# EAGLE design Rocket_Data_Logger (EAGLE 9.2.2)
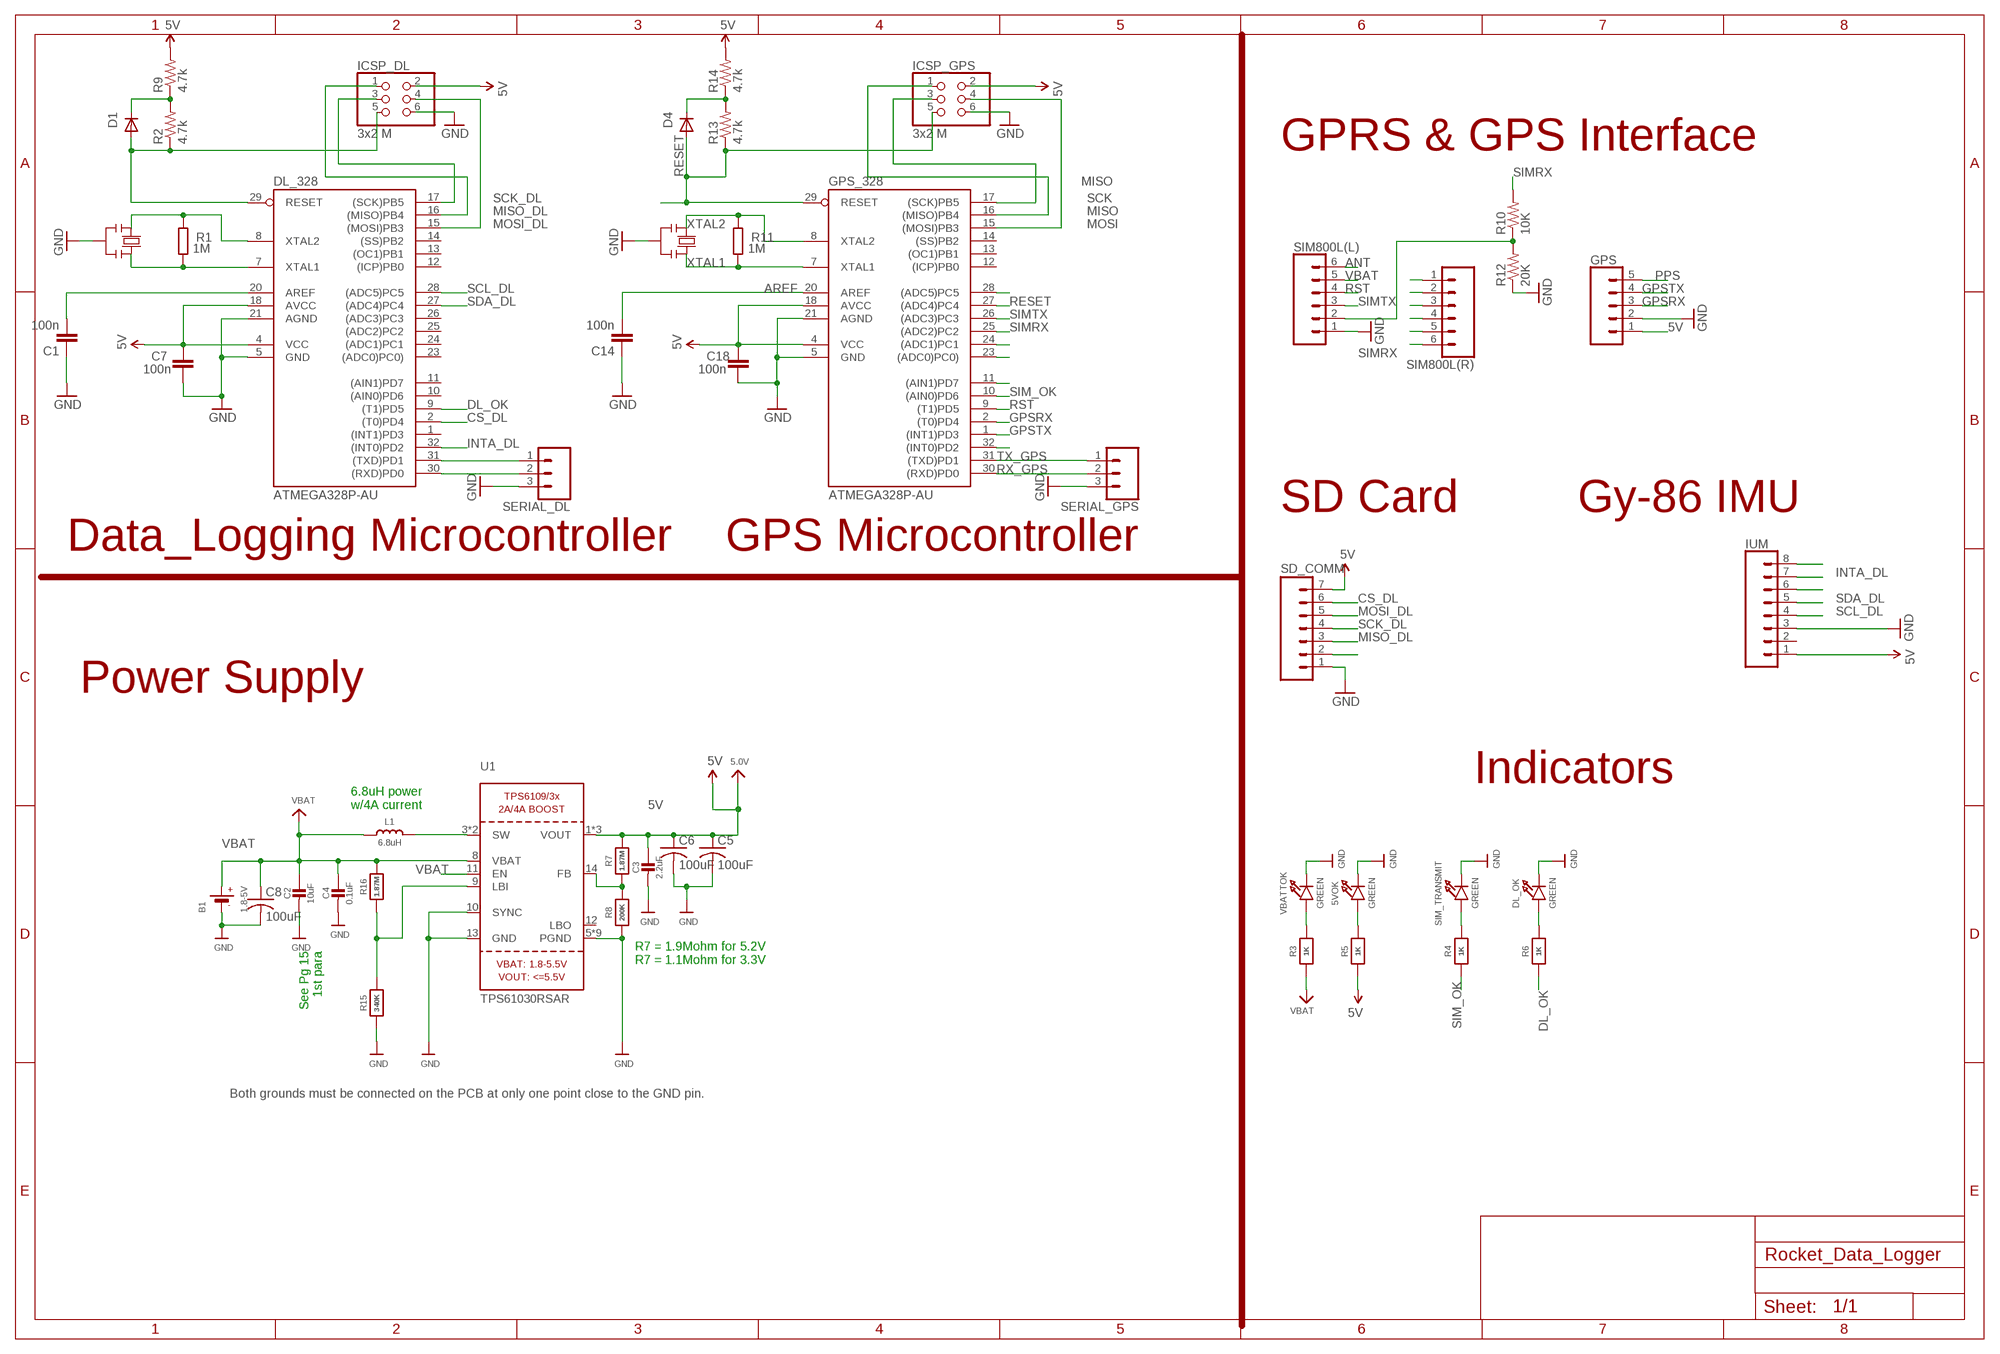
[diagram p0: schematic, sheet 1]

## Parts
5VOK  GREEN  LED0805_NOOUTLINE  [CHIPLED_0805_NOOUTLINE]
B1  1.8-5V  BATTERY  [JSTPH2]
C1  100n  C-EUC0805  [C0805]
C2  10uF  CAP_CERAMIC0805-NOOUTLINE  [0805-NO]
C3  2.2uF  CAP_CERAMIC0805-NOOUTLINE  [0805-NO]
C4  0.1uF  CAP_CERAMIC0805-NOOUTLINE  [0805-NO]
C5  100uF  C-USC1210  [C1210]
C6  100uF  C-USC1210  [C1210]
C7  100n  C-EUC0805  [C0805]
C8  100uF  C-USC1210  [C1210]
C14  100n  C-EUC0805  [C0805]
C18  100n  C-EUC0805  [C0805]
D1  DIODE-MINIMELF  [MINIMELF]
D4  DIODE-MINIMELF  [MINIMELF]
DL_328  ATMEGA328P-AU  [TQFP32-08]
DL_OK  GREEN  LED0805_NOOUTLINE  [CHIPLED_0805_NOOUTLINE]
GPS  CONN_05  [1X05]
GPS_328  ATMEGA328P-AU  [TQFP32-08]
ICSP_DL  3x2 M  PINHD-2X3  [2X03]
ICSP_GPS  3x2 M  PINHD-2X3  [2X03]
IUM  CONN_08"  [1X08]
L1  6.8uH  INDUCTOR-8X8  [INDUCTOR_8X8MM]
R1  1M  R-EU_R0805  [R0805]
R2  4.7k  4.7KOHM1/10W1%(0603)  [0603@1]
R3  1K  RESISTOR0805_NOOUTLINE  [0805-NO]
R4  1K  RESISTOR0805_NOOUTLINE  [0805-NO]
R5  1K  RESISTOR0805_NOOUTLINE  [0805-NO]
R6  1K  RESISTOR0805_NOOUTLINE  [0805-NO]
R7  1.87M  RESISTOR_0805MP  [_0805MP]
R8  200K  RESISTOR0805_NOOUTLINE  [0805-NO]
R9  4.7k  4.7KOHM1/10W1%(0603)  [0603@1]
R10  10K  RESISTOR0805-RES  [0805]
R11  1M  R-EU_R0805  [R0805]
R12  20K  RESISTOR0805-RES  [0805]
R13  4.7k  4.7KOHM1/10W1%(0603)  [0603@1]
R14  4.7k  4.7KOHM1/10W1%(0603)  [0603@1]
R15  340K  RESISTOR_0805MP  [_0805MP]
R16  1.87M  RESISTOR_0805MP  [_0805MP]
SD_COMM  M07  [1X07]
SERIAL_DL  CONN_03  [1X03]
SERIAL_GPS  CONN_03  [1X03]
SIM800L(L)  CONN_06SILK_FEMALE_PTH  [1X06]
SIM800L(R)  CONN_06SILK_FEMALE_PTH  [1X06]
SIM_TRANSMIT  GREEN  LED0805_NOOUTLINE  [CHIPLED_0805_NOOUTLINE]
U1  TPS61030RSAR  VREG_TPS6103X  [PVQFN-16]
VBATTOK  GREEN  LED0805_NOOUTLINE  [CHIPLED_0805_NOOUTLINE]
Y1  RESONATORMU  [RESONATOR]
Y2  RESONATORMU  [RESONATOR]

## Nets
5V: C3.1 C5.1 C6.1 C7.2 C18.2 DL_328.4(VCC) DL_328.18(AVCC) GPS.1 GPS_328.4(VCC) GPS_328.18(AVCC) ICSP_DL.2 ICSP_GPS.2 IUM.1 R5.1 R7.2 R9.2 R14.2 SD_COMM.7 U1.1(VOUT) U1.15(VOUT) U1.16(VOUT) ; supply symbol labelled 5.0V
ANT: SIM800L(L).6
AREF [aref]: C14.2 GPS_328.20(AREF)
CS_DL: DL_328.2((T0)PD4) SD_COMM.6
DL_OK: DL_328.9((T1)PD5) R6.1
FPS_RX: R10.1 R12.2 SIM800L(L).2
GND: 5VOK.C B1.1(-) C1.1 C2.2 C3.2 C4.2 C5.2 C6.2 C7.1 C8.2 C14.1 C18.1 DL_328.5(GND) DL_328.21(AGND) DL_OK.C GPS.2 GPS_328.5(GND) GPS_328.21(AGND) ICSP_DL.6 ICSP_GPS.6 IUM.3 R8.1 R12.1 R15.1 SD_COMM.1 SERIAL_DL.3 SERIAL_GPS.3 SIM800L(L).1 SIM_TRANSMIT.C U1.5(PGND) U1.6(PGND) U1.7(PGND) U1.10(SYNC) U1.13(GND) U1.P$18(PGND) U1.P$19(PGND) U1.P$20(PGND) U1.P$21(PGND) U1.P$22(PGND) U1.THERMAL(PGND) VBATTOK.C Y1.2 Y2.2
GPSRX: GPS.3 GPS_328.2((T0)PD4)
GPSTX: GPS.4 GPS_328.1((INT1)PD3)
INTA_DL: DL_328.32((INT0)PD2) IUM.7
MISO: GPS_328.16((MISO)PB4) ICSP_GPS.1
MISO_DL: DL_328.16((MISO)PB4) ICSP_DL.1 SD_COMM.3
MOSI: GPS_328.15((MOSI)PB3) ICSP_GPS.4
MOSI_DL: DL_328.15((MOSI)PB3) ICSP_DL.4 SD_COMM.5
N$1: D1.C R2.2 R9.1
N$2: DL_328.8(XTAL2) R1.2 Y1.1
N$3: L1.P$2 U1.3(SW) U1.4(SW)
N$4: IUM.6
N$5: D1.A DL_328.29(RESET) ICSP_DL.5 R2.1
N$6: IUM.8
N$7: R15.2 R16.1 U1.9(LBI)
N$9: R7.1 R8.2 U1.14(FB)
N$11: 5VOK.A R5.2
N$12: GPS_328.32((INT0)PD2)
N$13: DL_328.7(XTAL1) R1.1 Y1.3
N$14: C1.2 DL_328.20(AREF)
N$15: DL_328.31((TXD)PD1) SERIAL_DL.1
N$17: GPS_328.11((AIN1)PD7)
N$18: D4.C R13.2 R14.1
N$19: SD_COMM.2
N$20: DL_328.30((RXD)PD0) SERIAL_DL.2
N$21: R3.2 VBATTOK.A
N$22: SIM800L(R).1
N$23: SIM800L(R).2
N$24: SIM800L(R).3
N$25: SIM800L(R).4
N$26: SIM800L(R).5
N$27: SIM800L(R).6
N$28: R4.2 SIM_TRANSMIT.A
N$29: GPS_328.23((ADC0)PC0))
N$30: GPS_328.24((ADC1)PC1)
N$31: DL_OK.A R6.2
N$34: GPS_328.28((ADC5)PC5)
PPS: GPS.5
RESET: D4.A GPS_328.27((ADC4)PC4) GPS_328.29(RESET) ICSP_GPS.5 R13.1
RST: GPS_328.9((T1)PD5) SIM800L(L).4
RX_GPS: GPS_328.30((RXD)PD0) SERIAL_GPS.2
SCK: GPS_328.17((SCK)PB5) ICSP_GPS.3
SCK_DL: DL_328.17((SCK)PB5) ICSP_DL.3 SD_COMM.4
SCL_DL: DL_328.28((ADC5)PC5) IUM.4
SDA_DL: DL_328.27((ADC4)PC4) IUM.5
SIM_OK: GPS_328.10((AIN0)PD6) R4.1
SIMRX: GPS_328.25((ADC2)PC2) R10.2
SIMTX: GPS_328.26((ADC3)PC3) SIM800L(L).3
TX_GPS: GPS_328.31((TXD)PD1) SERIAL_GPS.1
VBAT: B1.2(+) C2.1 C4.1 C8.1 L1.P$1 R3.1 R16.2 SIM800L(L).5 U1.8(VBAT) U1.11(EN)
XTAL1: GPS_328.7(XTAL1) R11.1 Y2.3
XTAL2: GPS_328.8(XTAL2) R11.2 Y2.1
Unconnected: DL_328.1((INT1)PD3) DL_328.10((AIN0)PD6) DL_328.11((AIN1)PD7) DL_328.12((ICP)PB0) DL_328.13((OC1)PB1) DL_328.14((SS)PB2) DL_328.23((ADC0)PC0)) DL_328.24((ADC1)PC1) DL_328.25((ADC2)PC2) DL_328.26((ADC3)PC3) GPS_328.12((ICP)PB0) GPS_328.13((OC1)PB1) GPS_328.14((SS)PB2) IUM.2 U1.12(LBO)

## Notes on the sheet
- GPRS & GPS Interface
- SD Card | Gy-86 IMU
- Data_Logging Microcontroller | GPS Microcontroller
- Power Supply
- Indicators
- 6.8uH power
  w/4A current
- See Pg 15
  1st para
- R7 = 1.9Mohm for 5.2V
  R7 = 1.1Mohm for 3.3V
- Both grounds must be connected on the PCB at only one point close to the GND pin.

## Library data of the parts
5VOK DL_OK SIM_TRANSMIT VBATTOK = microbuilder:LED: LED
B1 = microbuilder:BATTERY: CR1220 SMT - Digikey: 3001K-ND
C1 C7 C14 C18 = SmartPrj:C-EU: CAPACITOR, European symbol
C2-C4 = microbuilder:CAP_CERAMIC: Ceramic Capacitors
C5 C6 C8 = rcl:C-US: CAPACITOR, American symbol
D1 D4 = diode:DIODE-: DIODE
DL_328 GPS_328 = SmartPrj:ATMEGA328P-: MICROCONTROLLER 4 Kbytes FLASH 128 bytes SRAM 256 bytes EEPROM UART 6-channel 10 bit ADC
GPS = SparkFun-Connectors:CONN_05: Multi connection point. Often used as Generic Header-pin footprint for 0.1 inch spaced/style header connections On any of the 0.1 inch spaced packages, you can populate with these: Break Away Headers - Straight (PRT-00116) Break Away Male Headers - Right Angle (PRT-00553) Female Headers (PRT-00115)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
ICSP_DL ICSP_GPS = SmartPrj:PINHD-2X3: PIN HEADER
IUM = SparkFun-Connectors:CONN_08: Multi connection point. Often used as Generic Header-pin footprint for 0.1 inch spaced/style header connections On any of the 0.1 inch spaced packages, you can populate with these: Break Away Headers - Straight (PRT-00116) Break Away Male Headers - Right Angle (PRT-00553) Female Headers (PRT-00115)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; PROD_ID: CONN-08438
L1 = microbuilder:INDUCTOR: Inductors
R1 R11 = SmartPrj:R-EU_: RESISTOR, European symbol
R2 R9 R13 R14 = SparkFun-Resistors:4.7KOHM1/10W1%(0603): RES-07857; PROD_ID: RES-07857
R3-R8 R15 R16 = microbuilder:RESISTOR: Resistors
R10 R12 = SparkFun:RESISTOR: Resistor
SD_COMM = SparkFun-Connectors:M07: Header 7 Standard 7-pin 0.1" header. Use with straight break away headers (SKU : PRT-00116), right angle break away headers (PRT-00553), swiss pins (PRT-00743), machine pins (PRT-00117), and female headers (PRT-00115). NOTES ON THE VARIANTS LOCK and LOCK_LONGPADS... This footprint was designed to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
SERIAL_DL SERIAL_GPS = SparkFun-Connectors:CONN_03: Multi connection point. Often used as Generic Header-pin footprint for 0.1 inch spaced/style header connections On any of the 0.1 inch spaced packages, you can populate with these: Break Away Headers - Straight (PRT-00116) Break Away Male Headers - Right Angle (PRT-00553) Female Headers (PRT-00115)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
SIM800L(L) SIM800L(R) = SparkFun-Connectors:CONN_06: Multi connection point. Often used as Generic Header-pin footprint for 0.1 inch spaced/style header connections On any of the 0.1 inch spaced packages, you can populate with these: Break Away Headers - Straight (PRT-00116) Break Away Male Headers - Right Angle (PRT-00553) Female Headers (PRT-00115)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; PROD_ID: CONN-08437
U1 = microbuilder:VREG_TPS6103X: TPS6103x 4A Boost - 1.8-5.5V Input, Adjustable Output to 5.5V
Y1 Y2 = SmartPrj:RESONATOR

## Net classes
0 default: width 0.152 mm, drill 0.305 mm, clearance 0.152 mm
3 usbvcc: width 0.508 mm, drill 0.61 mm, clearance 0.254 mm
4 aref: width 0.406 mm, drill 0.61 mm, clearance 0.254 mm

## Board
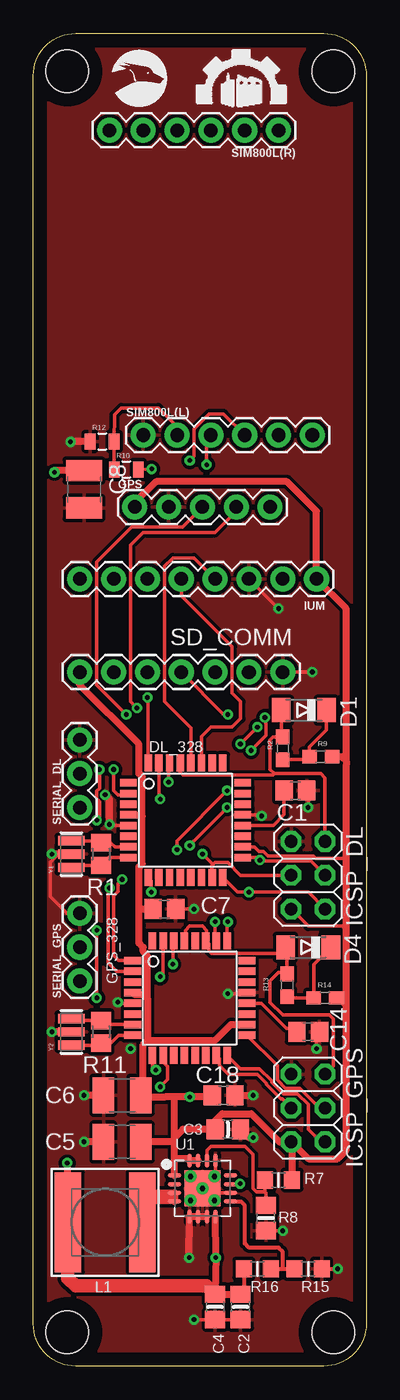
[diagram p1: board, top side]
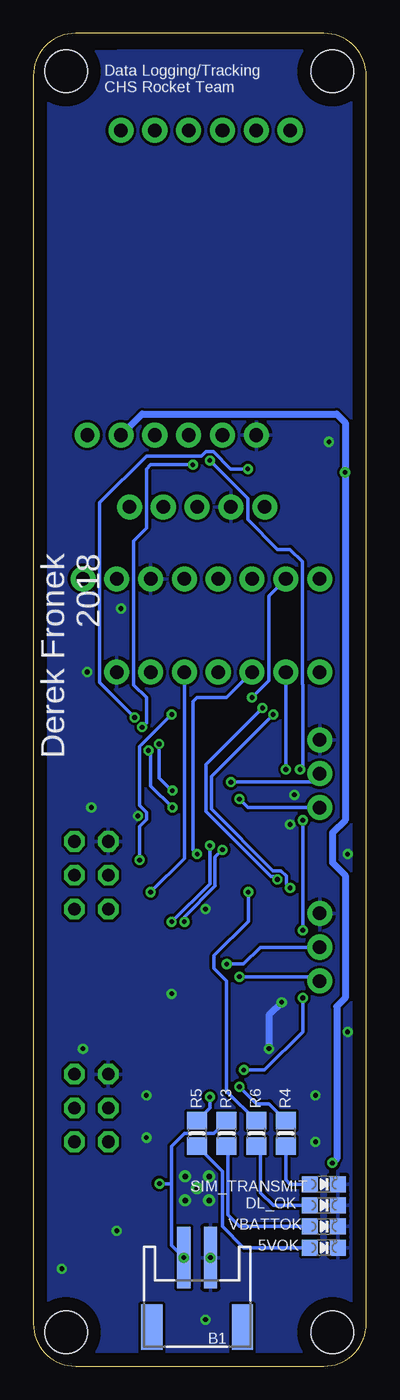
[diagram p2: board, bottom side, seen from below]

Size 25 x 99.99 mm. Coordinates in mm from the lower left corner, seen from the top.
Outline: 25,96.81 25,3.17 arc-90 21.82,0 3.17,0 arc-90 0,3.17 0,96.81 arc-90 3.17,99.99 21.82,99.99 arc-90 25,96.81
Copper layers (1*16): Top 0.035mm / dielectric 1.5mm / Bottom 0.035mm
Design rules "default": minimum track width 6mil, minimum drill 0.35mm, track to track 6mil, track to pad 6mil, pad to pad 6mil, via to via 6mil, smd to smd 6mil, copper to edge 40mil, drill to drill 6mil, minimum pad ring 10mil, minimum via ring 8mil, stop-mask expansion 4mil, vias tented up to drill 0mil, thermal gap 10mil
Holes 3.2 mm at 22.54,97.16 2.54,2.54 2.54,97.16 22.54,2.54

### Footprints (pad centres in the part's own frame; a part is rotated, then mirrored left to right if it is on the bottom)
CHIPLED_0805_NOOUTLINE = smd 1.2 x 1.2: A 0,-1.05; C 0,1.05
JSTPH2 = smd 1 x 4.6: 1 -1,-3.7; 2 1,-3.7 | smd 1.6 x 3.4: NC1 -3.4,1.5; NC2 3.4,1.5
C0805 = smd 1.3 x 1.5: 1 -0.85,0; 2 0.85,0
0805-NO = smd 1.3 x 1.5: 1 -0.95,0; 2 0.95,0
C1210 = smd 1.6 x 2.7: 1 -1.4,0; 2 1.4,0
MINIMELF = smd 1.4 x 1.8: A 1.7,0; C -1.7,0
TQFP32-08 = smd 1.27 x 0.559: 1 -4.293,2.8; 2 -4.293,2; 3 -4.293,1.2; 4 -4.293,0.4; 5 -4.293,-0.4; 6 -4.293,-1.2; 7 -4.293,-2; 8 -4.293,-2.8; 17 4.293,-2.8; 18 4.293,-2; 19 4.293,-1.2; 20 4.293,-0.4; 21 4.293,0.4; 22 4.293,1.2; 23 4.293,2; 24 4.293,2.8 | smd 0.559 x 1.27: 9 -2.8,-4.293; 10 -2,-4.293; 11 -1.2,-4.293; 12 -0.4,-4.293; 13 0.4,-4.293; 14 1.2,-4.293; 15 2,-4.293; 16 2.8,-4.293; 25 2.8,4.293; 26 2,4.293; 27 1.2,4.293; 28 0.4,4.293; 29 -0.4,4.293; 30 -1.2,4.293; 31 -2,4.293; 32 -2.8,4.293
1X05 = drill 1.016 pad 1.88: 1 0,0; 2 2.54,0; 3 5.08,0; 4 7.62,0; 5 10.16,0
2X03 = drill 0.95 pad 1.55 octagon: 1 -2.54,-1.27; 2 -2.54,1.27; 3 0,-1.27; 4 0,1.27; 5 2.54,-1.27; 6 2.54,1.27
1X08 = drill 1.016 pad 1.88: 1 0,0; 2 2.54,0; 3 5.08,0; 4 7.62,0; 5 10.16,0; 6 12.7,0; 7 15.24,0; 8 17.78,0
INDUCTOR_8X8MM = smd 2 x 7.5: P$1 -2.8,0; P$2 2.8,0
R0805 = smd 1.3 x 1.5: 1 -0.85,0; 2 0.85,0
0603@1 = smd 1.1 x 1: 1 -0.85,0; 2 0.85,0
_0805MP = smd 1.2 x 1.3: 1 -1.016,0; 2 1.016,0
0805 = smd 0.8 x 1.2: 1 -0.9,0; 2 0.9,0
1X07 = drill 1.016 pad 1.88: 1 0,0; 2 2.54,0; 3 5.08,0; 4 7.62,0; 5 10.16,0; 6 12.7,0; 7 15.24,0
1X03 = drill 1.016 pad 1.88: 1 0,0; 2 2.54,0; 3 5.08,0
1X06 = drill 1.016 pad 1.88: 1 0,0; 2 2.54,0; 3 5.08,0; 4 7.62,0; 5 10.16,0; 6 12.7,0
PVQFN-16 = smd 1.05 x 0.35: 1 -2.1,0.975; 2 -2.1,0.325; 3 -2.1,-0.325; 4 -2.1,-0.975; 9 2.1,-0.975; 10 2.1,-0.325; 11 2.1,0.325; 12 2.1,0.975 | smd 0.35 x 1.05: 5 -0.975,-2.1; 6 -0.325,-2.1; 7 0.325,-2.1; 8 0.975,-2.1; 13 0.975,2.1; 14 0.325,2.1; 15 -0.325,2.1; 16 -0.975,2.1 | drill 0.4: P$18 0,0; P$19 -0.9,0.9; P$20 0.9,0.9; P$21 0.9,-0.9; P$22 -0.9,-0.9 | smd 2.7 x 2.7: THERMAL 0,0
RESONATOR = smd 0.7 x 2: 1 -1,0; 2 0,0; 3 1,0

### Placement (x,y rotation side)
5VOK  3.17,8.89 270 bottom
B1  12.7,4.45 180 bottom
C1  19.68,43.18 180 top
C2  15.56,4.45 270 top
C3  14.61,17.78 0 top
C4  13.65,4.45 270 top
C5  6.67,16.83 180 top
C6  6.67,20.32 180 top
C7  9.84,34.29 180 top
C8  3.81,65.79 270 top
C14  20.64,25.08 180 top
C18  14.29,20.32 180 top
D1  20.32,49.21 180 top
D4  20.64,31.43 180 top
DL_328  11.43,40.96 0 top
DL_OK  3.17,12.06 270 bottom
GPS  7.62,64.45 0 top
GPS_328  11.75,27.62 0 top
ICSP_DL  20.64,36.83 90 top
ICSP_GPS  20.64,19.37 90 top
IUM  21.27,59.05 180 top
L1  5.4,10.79 0 top
R1  5.08,38.42 270 top
R2  18.73,46.35 270 top
R3  10.48,17.46 270 bottom
R4  6.03,17.46 270 bottom
R5  12.7,17.46 270 bottom
R6  8.26,17.46 270 bottom
R7  18.41,13.97 0 top
R8  17.46,11.11 90 top
R9  21.59,45.72 0 top
R10  6.98,67.27 0 top
R11  5.08,25.08 270 top
R12  5.17,69.38 0 top
R13  19.05,28.57 270 top
R14  21.91,27.62 0 top
R15  20.64,7.3 180 top
R16  16.83,7.3 180 top
SD_COMM  18.73,52.07 180 top
SERIAL_DL  3.49,41.91 90 top
SERIAL_GPS  3.49,28.89 90 top
SIM800L(L)  8.26,69.85 0 top
SIM800L(R)  18.41,92.71 180 top
SIM_TRANSMIT  3.17,13.65 270 bottom
U1  12.7,13.34 0 top
VBATTOK  3.17,10.48 270 bottom
Y1  2.86,38.42 90 top
Y2  2.86,25.08 90 top

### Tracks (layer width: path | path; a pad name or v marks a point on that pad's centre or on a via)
5V  (via drill 0.35)
  Top 0.254: 23.5,16.19 23.5,26.89 | 23.5,26.89 R14.2 | ICSP_DL.2 20.64,33.02 23.18,33.02 23.5,32.7 | 23.5,32.7 23.5,26.89 | 23.5,32.7 23.5,38.1 | 23.5,38.1 23.5,45.09 | DL_328.18 16.61,38.96 16.93,38.63 17.29,38.63 17.62,38.29 21.02,38.29 21.21,38.1 23.5,38.1
  Top 0.508: U1.1 10.6,15.56 | 10.6,15.56 10.6,16.83 | 10.6,16.83 10.6,17.14 | 10.6,17.14 10.6,20.2 | 10.6,17.14 11.23,17.78 C3.1 13.65,18.42 14.17,18.94 16.37,18.94 18.48,16.83 ICSP_GPS.2 | 10.6,16.83 C5.1 | 10.6,20.2 v11.75,20.2 13.24,20.2 C18.2 | 8.57,24.45 8.26,24.13 8.26,20.51 C6.1 8.22,20.17 9.85,20.17 9.88,20.2 10.6,20.2 | GPS_328.4 7.57,27.91 8.26,27.91 8.57,27.59 | 8.57,27.59 8.57,24.45 | ICSP_GPS.2 19.43,16.76 R7.2 | 10.6,15.56 11.6,15.56 U1.16 U1.15 | 8.57,24.45 13.65,24.45 14.83,25.62 GPS_328.18 | 8.57,27.59 8.57,30.79 8.26,31.11 8.26,31.43 7.94,31.75 7.94,34.29 | 8.18,41.27 8.18,37.71 7.94,37.47 7.94,34.29 | 8.18,41.27 8.18,44.2 7.94,44.45 7.94,46.67 3.49,51.12 SD_COMM.7 | DL_328.4 8.1,41.36 8.18,41.27 | 7.94,34.29 C7.2 | ICSP_GPS.2 20.64,15.56 22.86,15.56 23.5,16.19 23.5,45.09 23.5,45.4 | R9.2 23.18,45.72 23.5,45.4 | 23.5,45.4 23.5,56.83 IUM.1 21.27,64.14 19.05,66.36 9.21,66.36 7.62,64.77 GPS.1
  Bottom 0.254: R5.1 11.75,19.36 v11.75,20.2
AREF
  Top 0.254: GPS_328.20 17.14,27.22 19.01,25.36 19.51,25.36 C14.2
CS_DL  (via drill 0.35)
  Top 0.254: v6.03,44.77 6.03,43.18 6.35,42.86 7.04,42.86 DL_328.2
  Bottom 0.254: SD_COMM.6 v6.03,44.77
DL_OK  (via drill 0.35)
  Top 0.254: v8.86,35.57 8.86,36.44 DL_328.9
  Bottom 0.254: R6.1 10.48,20.64 10.48,28.89 11.43,29.84 11.43,30.8 8.86,33.37 v8.86,35.57
FPS_RX
  Top 0.254: R10.1 R12.2 6.09,71.37 6.6,71.88 9.4,71.88 10.79,70.48 SIM800L(L).2
GND  (via drill 0.35)
  Top 0.254: U1.13 13.68,14.31 U1.P$20 | R8.1 v18.73,10.16 | C2.2 C4.2 v12.07,3.5 v12.06,3.49 | U1.10 13.66,13.01 | 13.66,13.01 13.65,13.02 | U1.THERMAL 13.03,13.01 13.66,13.01 | C14.1 21.27,24.87 v21.27,23.81 | GPS_328.21 15.96,27.94 v14.61,27.94 | GPS_328.5 6.43,27.22 v6.35,27.3 | DL_328.21 17.06,41.36 v17.14,41.27 | C1.1 20.64,43.08 v20.64,41.91 | DL_328.5 5.8,40.56 v5.71,40.64 | C7.1 v12.06,34.29 | SERIAL_GPS.3 2.54,33.97 1.27,35.24 1.27,37.78 1.91,38.42 Y1.2 | SD_COMM.1 v20.95,52.07 | IUM.3 v18.41,56.83
  Top 0.305: R15.1 v22.86,7.3
  Top 0.508: B1.1 U1.5 U1.6 U1.7 | C5.2 v3.81,16.83 | C6.2 v3.81,20.32 | C3.2 16.19,17.14 v16.51,17.14 | C18.1 v16.51,20.32 | Y2.2 v1.39,25.08 | v5.71,40.64 5.71,42.55 v5.4,42.86 | R12.1 2.83,69.38 v2.79,69.34 | Y1.2 v1.39,38.42
  Bottom 0.254: v1.39,38.42 1.27,38.42
  Bottom 0.508: v1.39,25.08 1.27,25.08 | v6.35,27.3 7.3,26.35 v7.3,23.81
  other vias: 11.7,8.14
  pour Bottom (isolate 0.203): -9.78,-0.72 33.34,-0.84 32.71,98.6 -9.15,98.72
  pour Top (isolate 0.254): 0.64,99.06 24.13,99.06 24.45,0.95 0.95,0.95
GPSRX  (via drill 0.35)
  Top 0.254: GPS_328.2 6.25,29.62 5.63,30.25 5.63,35.79 | 5.63,35.79 5.63,35.88 | 5.63,35.79 v5.71,35.88 | v6.99,48.9 4.76,51.12 4.76,60.33 7.39,62.95 11.2,62.95 GPS.3
  Bottom 0.254: v5.71,35.88 6.01,36.17 6.01,36.78 6.39,37.17 7.01,37.17 11.63,41.79 11.63,44.25 v6.99,48.9
GPSTX  (via drill 0.35)
  Top 0.254: GPS_328.1 6.41,30.42 6.03,30.8 6.03,35.27 6.37,35.6 6.37,36.22 v6.67,36.51 | v7.79,49.38 7.62,49.21 7.62,49.53 7.3,49.85 7.3,61.59 8.26,62.55 13.65,62.55 15.24,64.14 GPS.4
  Bottom 0.254: v6.67,36.51 6.88,36.73 7.14,36.73 12.04,41.62 12.04,45.13 v7.79,49.38
INTA_DL  (via drill 0.35)
  Top 0.254: DL_328.32 8.63,50.11 v8.57,50.16
  Bottom 0.254: v8.57,50.16 7.3,51.44 7.3,57.78 IUM.7
MISO
  Top 0.254: GPS_328.16 15.56,22.31 17,22.31 17.91,21.4 17.91,21.3 18.76,20.45 19.84,20.45 20.64,19.65 20.64,17.78 21.59,16.83 ICSP_GPS.1
MISO_DL  (via drill 0.35)
  Top 0.254: DL_328.16 15.34,35.56 v16.19,35.56 20.64,35.56 ICSP_DL.1
  Bottom 0.254: SD_COMM.3 13.65,38.1 v16.19,35.56
MOSI
  Top 0.254: GPS_328.15 13.99,23.09 13.99,22.58 14.66,21.91 16.83,21.91 17.5,21.23 17.5,21.13 18.59,20.04 18.7,20.04 ICSP_GPS.4
MOSI_DL  (via drill 0.35)
  Top 0.254: DL_328.15 13.43,37.56 13.49,37.62 | 13.49,37.62 13.65,37.78 14.61,37.78 15.56,36.83 ICSP_DL.4 | v12.7,38.42 13.49,37.62
  Bottom 0.254: SD_COMM.5 10.48,50.16 12.7,50.16 13.02,49.85 13.02,38.73 v12.7,38.42
N$1
  Top 0.254: R9.1 20.52,45.51 R2.2 | D1.C 22.02,47.74 20.74,46.46 R9.1 | 20.74,45.62 R9.1
N$2
  Top 0.254: DL_328.8 5.67,38.16 R1.2 3.01,37.57 Y1.1
N$3
  Top 0.508: L1.P$2 8.25,12.39 | 8.25,12.39 8.26,12.7 8.57,12.7 | 8.57,12.7 8.26,13.02 U1.3 10.6,12.7 | 8.25,12.39 U1.4 10.6,12.7 | 10.6,12.7 8.57,12.7
N$5
  Top 0.254: D1.A 18.62,47.32 R2.1 18,47.2 17.78,46.99 17.78,44.77 18.1,44.45 | 18.1,44.45 21.59,44.45 21.91,44.13 ICSP_DL.5 | DL_328.29 11.03,44.53 11.23,44.34 17.98,44.34 18.1,44.45
N$7
  Top 0.305: U1.9 15.58,12.36 15.88,12.06 15.88,9.21 16.19,8.89 18.41,8.89 18.73,8.57 18.73,7.3 | R16.1 18.73,7.3 | 18.73,7.3 R15.2
N$9
  Top 0.254: U1.14 13.03,16.2 13.34,16.51 15.88,16.51 16.51,15.88 16.51,13.34 16.76,13.08 17.4,13.08 | 17.4,13.08 R7.1 | 17.4,13.08 17.46,13.02 17.46,12.38
  Top 0.305: 17.46,12.38 R8.2
N$11
  Bottom 0.254: 5VOK.A 9.21,8.89 10.79,10.48 10.79,14.61 R5.2
N$13
  Top 0.254: Y1.3 4.93,39.42 R1.1 5.82,39.27 6.13,38.96 DL_328.7
N$14
  Top 0.254: DL_328.20 18.02,40.56 18.84,41.38 C1.2
N$15  (via drill 0.35)
  Top 0.254: v9.53,42.55 9.43,42.64 DL_328.31
  Bottom 0.254: SERIAL_DL.1 8.89,41.91 v9.53,42.55
N$18
  Top 0.254: R13.2 19.15,27.62 R14.1 21.06,30.15 D4.C
N$20  (via drill 0.35)
  Top 0.254: v10.16,43.81 10.16,45.18 DL_328.30
  Bottom 0.254: SERIAL_DL.2 4.13,43.81 v10.16,43.81
N$21
  Bottom 0.254: VBATTOK.A 9.53,10.48 10.39,11.34 10.39,16.42 R3.2
N$28
  Bottom 0.254: R4.2 6.03,13.97 5.71,13.65 SIM_TRANSMIT.A
N$31
  Bottom 0.254: R6.2 7.94,16.2 7.94,13.02 6.99,12.06 DL_OK.A
RESET
  Top 0.254: ICSP_GPS.5 22.54,22.54 22.54,26.04 22.23,26.35 18.73,26.35 17.78,27.3 17.78,28.89 18.41,29.53 19.05,29.53 R13.1 19.05,31.11 | 19.05,31.11 19.05,31.32 D4.A | GPS_328.29 11.43,32 11.43,32.7 11.75,33.02 12.7,33.02 13.02,32.7 13.02,31.98 GPS_328.27 13.19,31.67 13.19,31.16 13.37,30.98 18.92,30.98 19.05,31.11
RST  (via drill 0.35)
  Top 0.254: v4.76,40.96 4.96,41.16 4.96,42.37 4.74,42.59 4.74,43.13 4.96,43.36 v4.96,44.77 | v4.76,32.7 v4.76,27.62 | v9.2,22.21 8.95,22.46 GPS_328.9 | SIM800L(L).4 14.29,71.44 13.2,71.44 12.06,70.3 12.06,68.26 v11.75,67.94
  Bottom 0.254: v4.96,44.77 4.76,44.97 4.76,51.12 4.81,51.17 4.81,60.38 5.71,61.28 6.67,61.28 8.89,63.5 8.89,65.09 v11.75,67.94 | v4.76,40.96 v4.76,32.7 | v4.76,27.62 4.76,25.08 7.63,22.21 v9.2,22.21
RX_GPS  (via drill 0.35)
  Top 0.254: v10.48,30.16 10.48,31.84 GPS_328.30
  Bottom 0.254: SERIAL_GPS.2 7.94,31.43 9.21,30.16 v10.48,30.16
SCK
  Top 0.254: ICSP_GPS.3 21.5,19.37 20.01,20.85 18.93,20.85 18.31,21.47 18.31,22.55 GPS_328.17
SCK_DL  (via drill 0.35)
  Top 0.254: DL_328.17 16.83,38.16 v17.02,37.97 17.1,37.88 20.85,37.88 ICSP_DL.3 | SD_COMM.4 14.29,48.9 v14.61,48.9
  Bottom 0.254: v17.02,37.97 17.02,40.48 16.49,41 16.49,41.55 17.02,42.08 17.02,46.48 v14.61,48.9
SCL_DL
  Top 0.254: DL_328.28 11.83,47.86 9.84,49.85 9.84,60.01 10.48,60.64 12.06,60.64 IUM.4
SDA_DL
  Top 0.254: DL_328.27 12.63,47.24 13.34,47.94 14.92,47.94 15.56,48.58 15.56,49.85 14.92,50.48 14.92,53.98 11.11,57.78 IUM.5
SIM_OK  (via drill 0.35)
  Top 0.254: GPS_328.10 9.75,22.82 10.09,22.48 10.09,21.52 v9.53,20.95
  Bottom 0.254: v9.53,20.95 8.26,19.68 7.3,19.68 R4.1
SIMRX  (via drill 0.35)
  Top 0.254: GPS_328.25 14.55,33.28 v14.61,33.34 | v11.75,39.05 14.56,41.86 v14.56,41.91 | v17.39,48.67 17.39,48.31 17.48,48.22 17.48,47.31 v16.36,46.19 | v8.89,67.31 R10.2
  Bottom 0.254: v14.61,33.34 11.75,36.2 v11.75,39.05 | v14.56,41.91 16.19,43.55 16.19,46.02 v16.36,46.19 | v17.39,48.67 20,51.28 20,64.77 16.49,68.28 12.74,68.28 12.72,68.26 12.38,68.26 12.36,68.26 12.02,68.6 11.47,68.6 10.18,67.31 v8.89,67.31
SIMTX  (via drill 0.35)
  Top 0.254: GPS_328.26 13.65,32.01 v13.65,33.34 | v10.79,38.73 10.79,39.42 v14.56,43.18 | v15.56,46.67 v16.83,47.94 | v13.02,67.63 13.02,69.53 SIM800L(L).3
  Bottom 0.254: v13.65,33.34 13.65,33.72 11.34,36.03 11.34,38.19 v10.79,38.73 | v14.56,43.18 14.61,43.18 15.56,44.13 v15.56,46.67 | v16.83,47.94 16.51,48.26 16.51,50.16 17.46,51.12 17.46,61.91 16.51,62.87 16.51,67.31 16.19,67.63 v13.02,67.63
TX_GPS  (via drill 0.35)
  Top 0.254: v9.53,29.21 9.75,29.43 GPS_328.31
  Bottom 0.254: SERIAL_GPS.1 3.81,29.21 v9.53,29.21
VBAT  (via drill 0.35)
  Top 0.254: U1.11 15.5,13.66 v15.52,13.69
  Top 0.305: R16.2 15.81,5.65 C2.1
  Top 0.508: C2.1 C4.1 13.68,6.99 B1.2 U1.8 | 2.6,7.94 L1.P$1 | L1.P$1 1.91,11.49 | L1.P$1 2.6,15.18 v2.54,15.24 | C8.1 1.72,67.19 v1.59,67.06
  Top 1.016: 2.6,7.94 2.6,6.61 3.17,6.03 13.02,6.03 C4.1
  Bottom 0.254: R3.1 11.43,17.46 13.65,17.46 14.61,16.51 14.61,13.72 | B1.2 14.61,9.05 14.61,13.72 | v15.52,13.69 14.63,13.69 14.61,13.72
  Bottom 0.508: v2.54,15.24 2.22,15.56 2.22,26.99 1.59,27.62 1.59,36.83 2.54,37.78 2.54,40.01 1.59,40.96 v1.59,67.06 1.59,70.8 2.22,71.44 16.83,71.44 SIM800L(L).5
  other vias: 13.7,8.14
XTAL1
  Top 0.254: GPS_328.7 5.39,25.62 R11.1 3.01,25.93 Y2.3
XTAL2
  Top 0.254: GPS_328.8 6.41,24.82 5.82,24.23 R11.2 4.93,24.08 Y2.1

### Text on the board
bNames: Data Logging/Tracking / CHS Rocket Team | Derek Fronek / 2018

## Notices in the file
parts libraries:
SparkFun-Resistors: Licensing: CC v3.0 Share-Alike You are welcome to use this library for commercial purposes.
SparkFun-Connectors: Licensing: Creative Commons ShareAlike 4.0 International - https://creativecommons.org/licenses/by-sa/4.0
